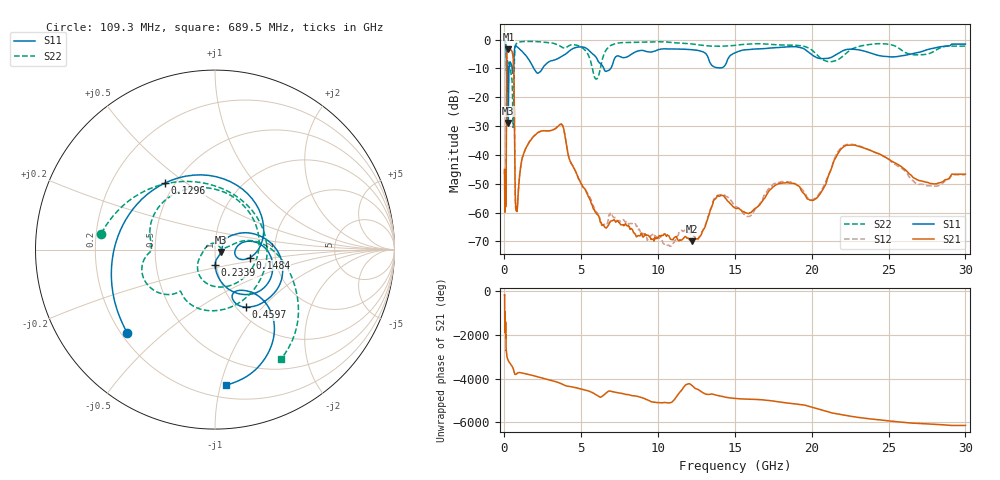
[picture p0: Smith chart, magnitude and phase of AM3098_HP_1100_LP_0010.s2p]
! Date/Time: Thu, Feb 28, 2019 8:44 AM
! Network Analyzer: Agilent Technologies E8364B Rev: A.07.50.67
! Sweep from 0.010 to 30.000 GHz, 1601 Points, Sweep Type: LOG
! Power Supply: 5.023 V, 0.002 A
# Hz S DB R 50
!freq MagS11 AngS11 MagS21 AngS21 MagS12 AngS12 MagS22 AngS22
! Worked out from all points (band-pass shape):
!   1601 points, 10 MHz to 30 GHz, reference 50 ohm
!   highest |S21| = -3.34 dB at 262.5 MHz (marker M1); lowest = -70.0 dB at 12.19 GHz (marker M2)
!   |S21| within 3 dB of the highest: 148.6 MHz to 566.8 MHz (418.2 MHz wide, 117 % of centre)
!   lowest |S11| = -28.9 dB at 246 MHz (marker M3), VSWR 1.07, Z = 53.4 - j1.43 ohm
!   |S11| at or under -10 dB: 204.6 MHz to 300.8 MHz (96.17 MHz wide, 38.1 % of centre); 1.909 GHz to 2.477 GHz (567.5 MHz wide, 25.9 % of centre); 6.47 GHz to 6.924 GHz (454.2 MHz wide, 6.78 % of centre)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
!   |S22| runs from -30.5 to -0.5 dB; largest |S21 - S12| = 0.01
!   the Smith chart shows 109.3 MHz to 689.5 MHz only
!   S11 on the Smith chart (normalised r, x): 109.3 MHz: 0.22, -0.38; 129.6 MHz: 0.44, +0.42; 148.4 MHz: 1.47, -0.14; 233.9 MHz: 0.99, -0.17; 459.7 MHz: 1.10, -0.81; 689.5 MHz: 0.29, -1.04
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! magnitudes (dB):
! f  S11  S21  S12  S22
! 10 MHz  -0.4  -46.6  -45.1  -0.5
! 38.04 MHz  -0.4  -58.5  -57.0  -0.7
! 109.3 MHz  -3.4  -54.9  -52.6  -3.9
! 129.6 MHz  -6.7  -21.4  -21.4  -10.6
! 144.7 MHz  -11.8  -7.5  -7.5  -9.5
! 148.4 MHz  -14.0  -6.4  -6.3  -9.9
! 233.9 MHz  -21.1  -3.4  -3.4  -8.8
! 246 MHz  -28.9  -3.4  -3.3  -9.0
! 262.5 MHz  -18.7  -3.3  -3.3  -9.0
! 459.7 MHz  -8.8  -3.9  -3.9  -13.0
! 550.5 MHz  -11.7  -5.5  -5.5  -28.8
! 617.6 MHz  -6.3  -13.5  -13.4  -13.7
! 689.5 MHz  -2.4  -49.0  -49.4  -2.9
! 821.5 MHz  -2.5  -58.9  -58.6  -1.2
! 2.084 GHz  -11.4  -32.7  -32.6  -0.7
! 3.723 GHz  -5.9  -29.4  -29.4  -2.6
! 5.989 GHz  -6.3  -60.4  -60.0  -13.7
! 7.926 GHz  -6.1  -64.5  -63.2  -1.0
! 12.19 GHz  -3.5  -70.0  -67.6  -1.5
! 20.2 GHz  -5.9  -55.4  -55.1  -4.6
! 22.56 GHz  -3.4  -36.6  -36.3  -3.5
! 30 GHz  -1.6  -46.7  -46.9  -2.3
